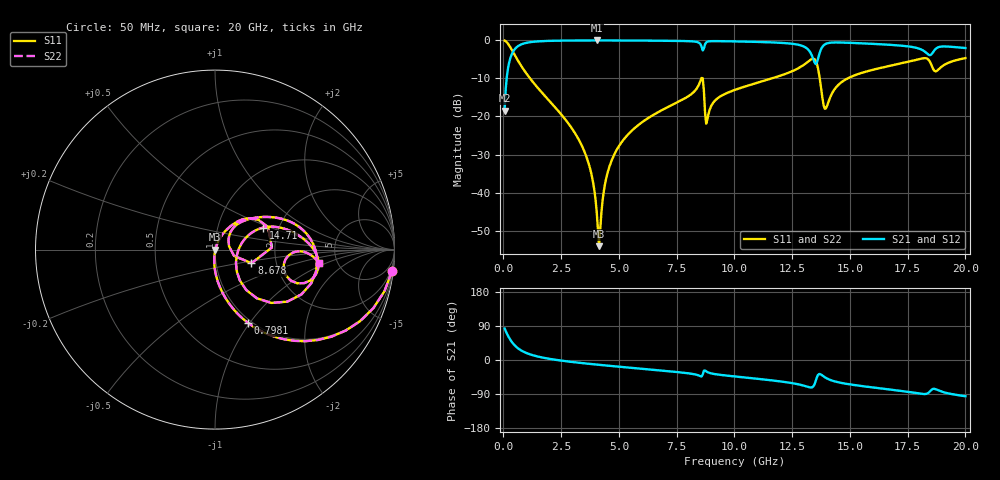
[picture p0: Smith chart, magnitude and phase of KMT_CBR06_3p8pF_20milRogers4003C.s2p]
! Data measured by Modelithics Inc. support@modelithics.com 813-866-6335
! KEMET CBR0603 3.8pF, Pad Width= 0.851mm, Pad Length= 0.64mm, Pad Gap= 0.62mm, 20mil Rogers 4003C substrate Data, January 2022
# hz S ma R 50
! 2 Port Network Data from SP1.SP block
! freq  magS11  angS11  magS21  angS21  magS12  angS12  magS22  angS22
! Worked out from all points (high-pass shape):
!   401 points, 50 MHz to 20 GHz, reference 50 ohm
!   highest |S21| = -0.02 dB at 4.04 GHz (marker M1); lowest = -18.5 dB at 50 MHz (marker M2)
!   |S21| within 3 dB of the highest: 412.4 MHz to 13.27 GHz (12.86 GHz wide, 188 % of centre); 13.71 GHz to 18.26 GHz (4.552 GHz wide, 28.5 % of centre)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
!   lowest |S11| = -54.1 dB at 4.14 GHz (marker M3), VSWR 1.00, Z = 50.2 - j0.0431 ohm
!   |S11| at or under -10 dB: 1.153 GHz to 8.569 GHz (7.417 GHz wide, 153 % of centre); 8.629 GHz to 11.62 GHz (2.988 GHz wide, 29.5 % of centre); 13.69 GHz to 14.9 GHz (1.208 GHz wide, 8.45 % of centre)
!   |S22| runs from -54.1 to -0.1 dB; largest |S21 - S12| = 0
!   S11 on the Smith chart (normalised r, x): 50 MHz: 1, -16; 798.1 MHz: 0.96, -0.98; 8.678 GHz: 1.49, -0.24; 14.71 GHz: 1.65, +0.44; 20 GHz: 3.62, -0.81
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5e7  0.9928 -7.0  0.1195 83.0  0.1195 83.0  0.9928 -7.0
2.99375e8  0.8096 -36.8  0.5862 53.1  0.5862 53.1  0.8096 -36.8
7.98125e8  0.4483 -65.7  0.8929 24.2  0.8929 24.2  0.4483 -65.7
3.391625e9  0.04142 -95.6  0.9972 -8.1  0.9972 -8.1  0.04142 -95.6
3.790625e9  0.01844 -94.7  0.9978 -10.6  0.9978 -10.6  0.01844 -94.7
4.04e9  0.005454 -81.2  0.9979 -12.1  0.9979 -12.1  0.005454 -81.2
4.13975e9  0.001973 -12.6  0.9979 -12.7  0.9979 -12.7  0.001973 -12.6
4.439e9  0.01489 67.6  0.9977 -14.5  0.9977 -14.5  0.01489 67.6
4.838e9  0.03343 69.5  0.9971 -16.8  0.9971 -16.8  0.03343 69.5
6.73325e9  0.1155 61.3  0.9903 -27.3  0.9903 -27.3  0.1155 61.3
8.52875e9  0.2937 34.3  0.8917 -42.7  0.8917 -42.7  0.2937 34.3
8.678375e9  0.2168 -20.4  0.7844 -28.2  0.7844 -28.2  0.2168 -20.4
8.828e9  0.09146 34.8  0.9598 -31.8  0.9598 -31.8  0.09146 34.8
1.0025e10  0.2238 45.3  0.9697 -43.5  0.9697 -43.5  0.2238 45.3
1.271825e10  0.4229 23.2  0.8821 -63.6  0.8821 -63.6  0.4229 23.2
1.336662e10  0.5724 -6.1  0.6185 -72.0  0.6185 -72.0  0.5724 -6.1
1.3616e10  0.4322 -43.4  0.5678 -39.6  0.5678 -39.6  0.4322 -43.4
1.391525e10  0.1262 -17.7  0.8861 -45.5  0.8861 -45.5  0.1262 -17.7
1.471325e10  0.2931 24.6  0.9356 -61.5  0.9356 -61.5  0.2931 24.6
1.670825e10  0.4612 10.9  0.8755 -77.7  0.8755 -77.7  0.4612 10.9
1.845388e10  0.5306 -20.6  0.6392 -83.5  0.6392 -83.5  0.5306 -20.6
2e10  0.5849 -7.3  0.7935 -95.6  0.7935 -95.6  0.5849 -7.3
